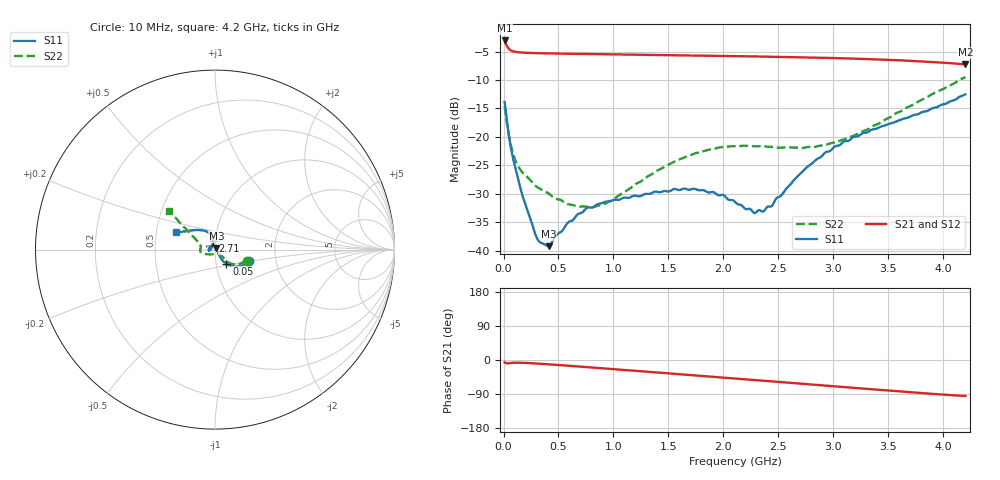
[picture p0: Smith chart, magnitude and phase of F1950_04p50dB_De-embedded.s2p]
! Integrated Device Technology
! Corporate Headquarters
! 6024 Silver Creek Valley Road
! San Jose, CA 95138  USA
! Phone:  1-408-284-8200
! Toll Free:  1-800-223-1366
! Webpage:  http://www.idt.com/
! Timing and RF Division
! 515 Groton Road, Suite 102
! Westford, MA 01886-6024
! Device:  F1950
! Description: 7-bit 0.25 dB Digital Step Attenuator
! Frequency:  150.0 -  4000.00 MHz
! Package:  4x4 mm Thin QFN Plastic Package: 24 pin
! Ports:  2 RF, 12 DC
!  Pin  1  = D0
!  Pin  2  = VDD
!  Pin  3  = Vmode
!  Pin  4  = GND
!  Pin  5  = RF1  =  Port 1
!  Pin  6  = GND
!  Pin  7  = GND
!  Pin  8  = GND
!  Pin  9  = GND
!  Pin 10  = GND
!  Pin 11  = GND
!  Pin 12  = GND
!  Pin 13  = GND
!  Pin 14  = RF2  =  Port 2
!  Pin 15  = GND
!  Pin 16  = LE
!  Pin 17  = CLK
!  Pin 18  = DATE
!  Pin 19  = D6
!  Pin 20  = D5
!  Pin 21  = D4
!  Pin 22  = D3
!  Pin 23  = D2
!  Pin 24  = D1
! State:  18
! Atten State:  4.50 dB
! Voltage:  +5.00 Volts
! Current:  Not Measured mA
! Data:  The device was measured on a the F195X evaluation board which has
!  individual transmission lines to the RF pins.  Data was collected
!  using a calibrated network analyzer.  The evaluation board was
!  de-embedded using a TRL calibration technique.
!  The reference plane is the edge of the package pin.
! Misc:  Board 2019
!  Action Tracker AT0250
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# GHz S dB R 50
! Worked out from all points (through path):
!   420 points, 10 MHz to 4.2 GHz, reference 50 ohm
!   highest |S21| = -3.06 dB at 10 MHz (marker M1); lowest = -7.3 dB at 4.2 GHz (marker M2)
!   group delay of S21, straight-line fit = 61.6 ps
!   lowest |S11| = -39.2 dB at 410 MHz (marker M3), VSWR 1.02, Z = 50.8 + j0.741 ohm
!   |S11| at or under -10 dB: start of sweep to end of sweep
!   |S22| runs from -32.4 to -9.5 dB; largest |S21 - S12| = 0.00067
!   S11 on the Smith chart (normalised r, x): 10 MHz: 1.46, -0.20; 50 MHz: 1.12, -0.18; 2.71 GHz: 0.97, +0.09; 4.2 GHz: 0.63, +0.13
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0.01  -13.89 -18.7  -3.06 -5.8  -3.06 -5.8  -14.59 -19.2
0.05  -19.91 -50.8  -4.56 -8.4  -4.56 -8.4  -19.90 -44.0
0.09  -24.06 -55.9  -4.97 -7.3  -4.97 -7.3  -23.18 -44.0
0.13  -27.17 -53.9  -5.11 -7.1  -5.11 -7.1  -25.08 -43.0
0.29  -37.15 -15.3  -5.29 -9.1  -5.28 -9.1  -28.59 -45.9
0.33  -38.51 0.8  -5.30 -9.8  -5.30 -9.8  -29.08 -47.5
0.41  -39.21 41.7  -5.34 -11.4  -5.33 -11.4  -29.93 -49.0
0.58  -35.18 88.6  -5.38 -14.9  -5.38 -14.9  -31.81 -60.4
0.71  -33.34 106.1  -5.42 -17.7  -5.42 -17.7  -32.25 -74.8
0.93  -31.38 126.5  -5.47 -22.6  -5.47 -22.6  -31.70 -104.0
1.41  -29.71 168.6  -5.60 -33.2  -5.60 -33.3  -25.79 -149.6
1.74  -29.13 -173.6  -5.69 -40.6  -5.69 -40.7  -22.91 -163.8
2  -30.21 -173.1  -5.77 -46.5  -5.77 -46.6  -21.79 -171.4
2.11  -31.51 -177.3  -5.81 -49.0  -5.81 -49.0  -21.65 -174.2
2.28  -33.40 158.4  -5.86 -52.8  -5.86 -52.9  -21.65 -178.0
2.36  -33.13 143.1  -5.89 -54.6  -5.89 -54.7  -21.62 -179.9
2.44  -32.14 126.2  -5.92 -56.4  -5.92 -56.4  -21.76 178.2
2.71  -26.27 102.8  -6.02 -62.6  -6.01 -62.6  -21.97 169.9
2.81  -24.60 100.9  -6.06 -64.9  -6.06 -64.9  -21.83 166.7
3.1  -20.76 107.0  -6.20 -71.6  -6.20 -71.6  -20.43 158.7
3.51  -17.69 124.2  -6.47 -80.9  -6.47 -80.9  -16.63 148.7
4.2  -12.53 156.0  -7.28 -95.0  -7.28 -95.0  -9.49 140.0
